| IBIS file stm32u595_599_5a5_5a9_wlcsp150_dsi_smps.ibs
[IBIS ver] 4.2
[File name] stm32u595_599_5a5_5a9_wlcsp150_dsi_smps.ibs
[File Rev] rev2.0
[Date]  11-09-2023
[Source] Data Created at STMicroelectronics
[Notes]  File originated from ELDO simulations.
[Disclaimer]  This information is for modeling purpose only and is
   not guaranteed. The information is subject to change without
   notice.
[Copyright] Copyright 2023 STMicroelectronics Inc.
|   Component stm32u595_599_5a5_5a9_wlcsp150_dsi_smps
[Component] stm32u595_599_5a5_5a9_wlcsp150_dsi_smps
[Manufacturer] STMicroelectronics
[Package]
| variable   typ   min   max
R_pkg  0  NA  NA
L_pkg  0  NA  NA
C_pkg  0  NA  NA
[Pin]   signal_name   model_name
A1  VDDUSB  power
A3  VDD  power
A5  PC12  io8_166m_hslv_ft
A7  VDD  power
A9  PB5  io8_166m_hslv_ft
A11  VDD  power
A13  PC14-OSC32_IN  nc
AA1  VSS  gnd
AA3  PB12  io8_166m_hslv_ft
AA5  PB11  io8_100m_hslv_ft
AA7  PE8  io8_100m_hslv_ft
AA9  PF13  io8_100m_hslv_ft
AA11  PA5  io8_100m_ft
AA13  VSSA_VREFM  nc
AB2  VDD11  nc
AB4  VDDSMPS  nc
AB6  PE13  io8_100m_hslv_ft
AB8  VSS  gnd
AB10  VSS  gnd
AB12  VREFP  nc
AC1  VDD  power
AC3  VSSSMPS  nc
AC5  VLXSMPS  nc
AC7  VDD  power
AC9  VDD  power
AC11  VDD  power
AC13  VDDA  nc
B2  VDD11  nc
B4  PA15  nc
B6  PD4  io8_100m_hslv_ft
B8  PB3  io8_100m_i2c_ft
B10  VDD11  nc
B12  PC15-OSC32_OUT  nc
C1  PA12  io8_100m_ft
C3  VSS  gnd
C5  PD0  io8_100m_hslv_ft
C7  VSS  gnd
C9  PB8  io8_100m_i2c_ft
C11  VSS  gnd
C13  VBAT  power
D2  VSS  gnd
D4  PC10  io8_100m_ft
D6  PD5  io8_100m_hslv_ft
D8  PB6  io8_100m_i2c_ft
D10  PE2  io8_100m_hslv_ft
D12  PE6  io8_100m_hslv_tamp_ft
E1  PA11  io8_100m_ft
E3  PA13  io8_100m_ft
E5  PD1  io8_100m_hslv_ft
E7  PB4  io8_100m_i2c_ft
E9  PE1  io8_100m_hslv_ft
E11  PC13  io8_100m_ft
E13  DSI_D0P  nc
F2  PA9  io8_100m_usb_vbus_ft
F4  PA14  io8_100m_ft
F6  PD6  io8_166m_hslv_ft
F8  PB9  io8_100m_i2c_ft
F10  PE5  io8_100m_hslv_tamp_ft
F12  PF2  io8_100m_hslv_ft
G1  VDDIO2  power
G3  PA10  io8_100m_usb_id
G5  PD2  io8_100m_ft
G7  PB7  io8_spi_hslv_ft
G9  PE3  io8_100m_hslv_tamp_ft
G11  PF0  io8_100m_hslv_ft
G13  DSI_D0N  nc
H2  VSS  gnd
H4  PA8  io8_166m_hslv_ft
H6  PD7  io8_100m_hslv_ft
H8  PE0  io8_100m_hslv_ft
H10  PF1  io8_100m_hslv_ft
H12  VDDDSI  nc
J1  PG7  io8_100m_hslv_ft
J3  PC7  io8_100m_ft
J5  PC11  io8_100m_hslv_ft
J7  PH3-BOOT0  nc
J9  PE4  io8_100m_hslv_tamp_ft
J11  PF6  io8_100m_hslv_ft
J13  DSI_CKP  nc
K2  PG8  io8_100m_i2c_ft
K4  PC8  io8_100m_ft
K6  PD3  io8_166m_hslv_ft
K8  PF10  io8_166m_hslv_ft
K10  PF7  io8_100m_hslv_ft
K12  VSSDSI  nc
L1  PG3  io8_100m_hslv_ft
L3  PG5  io8_100m_hslv_ft
L5  PC9  io8_100m_ft
L7  PC1  io8_spi_hslv_ft
L9  PF9  io8_100m_hslv_ft
L11  PF3  io8_100m_hslv_ft
L13  DSI_CKN  nc
M2  PG4  io8_100m_hslv_ft
M4  PG6  io8_100m_hslv_ft
M6  PB2  io8_100m_hslv_tamp_ft
M8  PA4  io8_100m_hslv_ft
M10  PF8  io8_100m_hslv_ft
M12  VDD11DSI  nc
N1  PG2  io8_100m_hslv_ft
N3  PD13  io8_100m_hslv_ft
N5  PC6  io8_100m_ft
N7  PC5  io8_100m_tamp_ft
N9  PA3  io8_166m_hslv_ft
N11  PF4  io8_spi_ft
N13  DSI_D1P  nc
P2  PD14  io8_100m_hslv_ft
P4  PE14  io8_100m_hslv_ft
P6  PG0  io8_100m_hslv_ft
P8  PA7  io8_100m_hslv_ft
P10  PC0  io8_100m_hslv_ft
P12  VSSDSI  nc
R1  PD15  io8_100m_hslv_ft
R3  PD11  io8_100m_hslv_ft
R5  PE10  io8_166m_hslv_ft
R7  PF11  io8_166m_hslv_ft
R9  PA2  io8_100m_hslv_ft
R11  PF5  io8_spi_ft
R13  DSI_D1N  nc
T2  PD12  io8_100m_hslv_ft
T4  PE15  io8_100m_hslv_ft
T6  PE7  io8_100m_hslv_ft
T8  PC4  io8_100m_hslv_ft
T10  PC3  io8_100m_hslv_ft
T12  VSS  gnd
U1  VDD  power
U3  PD9  io8_100m_hslv_ft
U5  PE11  io8_100m_hslv_ft
U7  PF15  io8_100m_hslv_ft
U9  PA6  io8_100m_hslv_ft
U11  NRST  nc
U13  VDD  power
V2  VSS  gnd
V4  PB14  io8_100m_i2c_ft
V6  PE9  io8_166m_hslv_ft
V8  PF12  io8_100m_hslv_ft
V10  PA1  io8_100m_hslv_tamp_ft
V12  PH1-OSC_OUT   nc
W1  PD10  io8_100m_hslv_ft
W3  PD8  io8_100m_hslv_ft
W5  PB10  io8_spi_hslv_ft
W7  PG1  io8_100m_hslv_ft
W9  PB1  io8_100m_hslv_ft
W11  PA0  io8_100m_hslv_tamp_ft
W13  PH0-OSC_IN  nc
Y2  PB15  nc
Y4  PB13  io8_100m_i2c_ft
Y6  PE12  io8_100m_hslv_ft
Y8  PF14  io8_100m_hslv_ft
Y10  PB0  io8_100m_hslv_ft
Y12  PC2  io8_100m_hslv_ft
[Package Model]   481-wlcsp-150-2rdl-dsi-220915
[Pin Mapping]   pulldown_ref   pullup_ref   | Comment
A1  nc  vddusb
A3  nc  vddiom
A5  gndio  vddiom
A7  nc  vddiom
A9  gndio  vddiom
A11  nc  vddiom
A13  nc  nc
AA1  gndio  nc
AA3  gndio  vddiom
AA5  gndio  vddiom
AA7  gndio  vddiom
AA9  gndio  vddiom
AA11  gndio  vddiom
AA13  nc  nc
AB2  nc  nc
AB4  nc  nc
AB6  gndio  vddiom
AB8  gndio  nc
AB10  gndio  nc
AB12  nc  nc
AC1  nc  vddiom
AC3  nc  nc
AC5  nc  nc
AC7  nc  vddiom
AC9  nc  vddiom
AC11  nc  vddiom
AC13  nc  nc
B2  nc  nc
B4  nc  nc
B6  gndio  vddiom
B8  gndio  vddiom
B10  nc  nc
B12  nc  nc
C1  gndio  vddiom  | Depending on IO usage
| C1  gndio  vddusb  | Depending on IO usage
C3  gndio  nc
C5  gndio  vddiom
C7  gndio  nc
C9  gndio  vddiom
C11  gndio  nc
C13  nc  vsw
D2  gndio  nc
D4  gndio  vddiom
D6  gndio  vddiom
D8  gndio  vddiom
D10  gndio  vddiom
D12  gndio  vddiom
E1  gndio  vddiom  | Depending on IO usage
| E1  gndio  vddusb  | Depending on IO usage
E3  gndio  vddiom  | Depending on IO usage
| E3  gndio  vddusb  | Depending on IO usage
E5  gndio  vddiom
E7  gndio  vddiom
E9  gndio  vddiom
E11  gndio  vddiom  | Depending on IO usage
| E11  gndio  vsw  | Depending on IO usage
E13  nc  nc
F2  gndio  vddiom  | Depending on IO usage
| F2  gndio  vddusb  | Depending on IO usage
F4  gndio  vddiom
F6  gndio  vddiom
F8  gndio  vddiom
F10  gndio  vddiom
F12  gndio  vddiom
G1  nc  vddio2
G3  gndio  vddiom  | Depending on IO usage
| G3  gndio  vddusb  | Depending on IO usage
G5  gndio  vddiom
G7  gndio  vddiom
G9  gndio  vddiom
G11  gndio  vddiom
G13  nc  nc
H2  gndio  nc
H4  gndio  vddiom
H6  gndio  vddiom
H8  gndio  vddiom
H10  gndio  vddiom
H12  nc  nc
J1  gndio  vddiom  | Depending on IO usage
| J1  gndio  vddio2  | Depending on IO usage
J3  gndio  vddiom
J5  gndio  vddiom
J7  nc  nc
J9  gndio  vddiom
J11  gndio  vddiom
J13  nc  nc
K2  gndio  vddiom  | Depending on IO usage
| K2  gndio  vddio2  | Depending on IO usage
K4  gndio  vddiom
K6  gndio  vddiom
K8  gndio  vddiom
K10  gndio  vddiom
K12  nc  nc
L1  gndio  vddiom  | Depending on IO usage
| L1  gndio  vddio2  | Depending on IO usage
L3  gndio  vddiom  | Depending on IO usage
| L3  gndio  vddio2  | Depending on IO usage
L5  gndio  vddiom
L7  gndio  vddiom
L9  gndio  vddiom
L11  gndio  vddiom
L13  nc  nc
M2  gndio  vddiom  | Depending on IO usage
| M2  gndio  vddio2  | Depending on IO usage
M4  gndio  vddiom  | Depending on IO usage
| M4  gndio  vddio2  | Depending on IO usage
M6  gndio  vddiom
M8  gndio  vddiom
M10  gndio  vddiom
M12  nc  nc
N1  gndio  vddiom  | Depending on IO usage
| N1  gndio  vddio2  | Depending on IO usage
N3  gndio  vddiom
N5  gndio  vddiom
N7  gndio  vddiom
N9  gndio  vddiom
N11  gndio  vddiom
N13  nc  nc
P2  gndio  vddiom
P4  gndio  vddiom
P6  gndio  vddiom
P8  gndio  vddiom
P10  gndio  vddiom
P12  nc  nc
R1  gndio  vddiom
R3  gndio  vddiom
R5  gndio  vddiom
R7  gndio  vddiom
R9  gndio  vddiom
R11  gndio  vddiom
R13  nc  nc
T2  gndio  vddiom
T4  gndio  vddiom
T6  gndio  vddiom
T8  gndio  vddiom
T10  gndio  vddiom
T12  gndio  nc
U1  nc  vddiom
U3  gndio  vddiom
U5  gndio  vddiom
U7  gndio  vddiom
U9  gndio  vddiom
U11  nc  nc
U13  nc  vddiom
V2  gndio  nc
V4  gndio  vddiom
V6  gndio  vddiom
V8  gndio  vddiom
V10  gndio  vddiom
V12  nc  nc
W1  gndio  vddiom
W3  gndio  vddiom
W5  gndio  vddiom
W7  gndio  vddiom
W9  gndio  vddiom
W11  gndio  vddiom
W13  nc  nc
Y2  nc  nc
Y4  gndio  vddiom
Y6  gndio  vddiom
Y8  gndio  vddiom
Y10  gndio  vddiom
Y12  gndio  vddiom
[Model Selector] io8_100m_ft
io8_100m_ft_hs_1v2  "IO8_FT 100MHz high speed @ 1.2V"
io8_100m_ft_fs_1v2  "IO8_FT 100MHz fast speed @ 1.2V"
io8_100m_ft_fs_pd_1v2  "IO8_FT 100MHz fast speed @ 1.2V pulldown"
io8_100m_ft_ms_1v2  "IO8_FT 100MHz med speed @ 1.2V"
io8_100m_ft_ms_pd_1v2  "IO8_FT 100MHz med speed @ 1.2V pulldown"
io8_100m_ft_ls_1v2  "IO8_FT 100MHz low speed @ 1.2V"
io8_100m_ft_ls_pd_1v2  "IO8_FT 100MHz low speed @ 1.2V pulldown"
io8_100m_ft_hs_1v8  "IO8_FT 100MHz high speed @ 1.8V"
io8_100m_ft_hs_pd_1v8  "IO8_FT 100MHz high speed @ 1.8V pulldown"
io8_100m_ft_fs_1v8  "IO8_FT 100MHz fast speed @ 1.8V"
io8_100m_ft_fs_pd_1v8  "IO8_FT 100MHz fast speed @ 1.8V pulldown"
io8_100m_ft_ms_1v8  "IO8_FT 100MHz med speed @ 1.8V"
io8_100m_ft_ms_pd_1v8  "IO8_FT 100MHz med speed @ 1.8V pulldown"
io8_100m_ft_ls_1v8  "IO8_FT 100MHz low speed @ 1.8V"
io8_100m_ft_ls_pd_1v8  "IO8_FT 100MHz low speed @ 1.8V pulldown"
io8_100m_ft_hs_3v3  "IO8_FT 100MHz high speed @ 3.3V"
io8_100m_ft_hs_pd_3v3  "IO8_FT 100MHz high speed @ 3.3V pulldown"
io8_100m_ft_fs_3v3  "IO8_FT 100MHz fast speed @ 3.3V"
io8_100m_ft_fs_pd_3v3  "IO8_FT 100MHz fast speed @ 3.3V pulldown"
io8_100m_ft_ms_3v3  "IO8_FT 100MHz med speed @ 3.3V"
io8_100m_ft_ms_pd_3v3  "IO8_FT 100MHz med speed @ 3.3V pulldown"
io8_100m_ft_ls_3v3  "IO8_FT 100MHz low speed @ 3.3V"
io8_100m_ft_ls_pd_3v3  "IO8_FT 100MHz low speed @ 3.3V pulldown"
[Model Selector] io8_100m_hslv_ft
io8_100m_ft_hs_1v2  "IO8_FT 100MHz high speed @ 1.2V"
io8_100m_ft_hs_pu_1v2  "IO8_FT 100MHz high speed @ 1.2V pullup"
io8_100m_ft_hs_pd_1v2  "IO8_FT 100MHz high speed @ 1.2V pulldown"
io8_100m_ft_fs_1v2  "IO8_FT 100MHz fast speed @ 1.2V"
io8_100m_ft_fs_pu_1v2  "IO8_FT 100MHz fast speed @ 1.2V pullup"
io8_100m_ft_fs_pd_1v2  "IO8_FT 100MHz fast speed @ 1.2V pulldown"
io8_100m_ft_ms_1v2  "IO8_FT 100MHz med speed @ 1.2V"
io8_100m_ft_ms_pu_1v2  "IO8_FT 100MHz med speed @ 1.2V pullup"
io8_100m_ft_ms_pd_1v2  "IO8_FT 100MHz med speed @ 1.2V pulldown"
io8_100m_ft_ls_1v2  "IO8_FT 100MHz low speed @ 1.2V"
io8_100m_ft_ls_pu_1v2  "IO8_FT 100MHz low speed @ 1.2V pullup"
io8_100m_ft_ls_pd_1v2  "IO8_FT 100MHz low speed @ 1.2V pulldown"
io8_100m_ft_hs_1v8  "IO8_FT 100MHz high speed @ 1.8V"
io8_100m_ft_hs_pu_1v8  "IO8_FT 100MHz high speed @ 1.8V pullup"
io8_100m_ft_hs_pd_1v8  "IO8_FT 100MHz high speed @ 1.8V pulldown"
io8_100m_ft_fs_1v8  "IO8_FT 100MHz fast speed @ 1.8V"
io8_100m_ft_fs_pu_1v8  "IO8_FT 100MHz fast speed @ 1.8V pullup"
io8_100m_ft_fs_pd_1v8  "IO8_FT 100MHz fast speed @ 1.8V pulldown"
io8_100m_ft_ms_1v8  "IO8_FT 100MHz med speed @ 1.8V"
io8_100m_ft_ms_pu_1v8  "IO8_FT 100MHz med speed @ 1.8V pullup"
io8_100m_ft_ms_pd_1v8  "IO8_FT 100MHz med speed @ 1.8V pulldown"
io8_100m_ft_ls_1v8  "IO8_FT 100MHz low speed @ 1.8V"
io8_100m_ft_ls_pu_1v8  "IO8_FT 100MHz low speed @ 1.8V pullup"
io8_100m_ft_ls_pd_1v8  "IO8_FT 100MHz low speed @ 1.8V pulldown"
io8_100m_ft_hs_3v3  "IO8_FT 100MHz high speed @ 3.3V"
io8_100m_ft_hs_pu_3v3  "IO8_FT 100MHz high speed @ 3.3V pullup"
io8_100m_ft_hs_pd_3v3  "IO8_FT 100MHz high speed @ 3.3V pulldown"
io8_100m_ft_fs_3v3  "IO8_FT 100MHz fast speed @ 3.3V"
io8_100m_ft_fs_pu_3v3  "IO8_FT 100MHz fast speed @ 3.3V pullup"
io8_100m_ft_fs_pd_3v3  "IO8_FT 100MHz fast speed @ 3.3V pulldown"
io8_100m_ft_ms_3v3  "IO8_FT 100MHz med speed @ 3.3V"
io8_100m_ft_ms_pu_3v3  "IO8_FT 100MHz med speed @ 3.3V pullup"
io8_100m_ft_ms_pd_3v3  "IO8_FT 100MHz med speed @ 3.3V pulldown"
io8_100m_ft_ls_3v3  "IO8_FT 100MHz low speed @ 3.3V"
io8_100m_ft_ls_pu_3v3  "IO8_FT 100MHz low speed @ 3.3V pullup"
io8_100m_ft_ls_pd_3v3  "IO8_FT 100MHz low speed @ 3.3V pulldown"
io8_100m_hslv_ft_hs_1v2  "IO8_FT 100MHz HSLV high speed @ 1.2V"
io8_100m_hslv_ft_hs_pu_1v2  "IO8_FT 100MHz HSLV high speed @ 1.2V pullup"
io8_100m_hslv_ft_hs_pd_1v2  "IO8_FT 100MHz HSLV high speed @ 1.2V pulldown"
io8_100m_hslv_ft_fs_1v2  "IO8_FT 100MHz HSLV fast speed @ 1.2V"
io8_100m_hslv_ft_fs_pu_1v2  "IO8_FT 100MHz HSLV fast speed @ 1.2V pullup"
io8_100m_hslv_ft_fs_pd_1v2  "IO8_FT 100MHz HSLV fast speed @ 1.2V pulldown"
io8_100m_hslv_ft_ms_1v2  "IO8_FT 100MHz HSLV med speed @ 1.2V"
io8_100m_hslv_ft_ms_pu_1v2  "IO8_FT 100MHz HSLV med speed @ 1.2V pullup"
io8_100m_hslv_ft_ms_pd_1v2  "IO8_FT 100MHz HSLV med speed @ 1.2V pulldown"
io8_100m_hslv_ft_ls_1v2  "IO8_FT 100MHz HSLV low speed @ 1.2V"
io8_100m_hslv_ft_ls_pu_1v2  "IO8_FT 100MHz HSLV low speed @ 1.2V pullup"
io8_100m_hslv_ft_ls_pd_1v2  "IO8_FT 100MHz HSLV low speed @ 1.2V pulldown"
io8_100m_hslv_ft_hs_1v8  "IO8_FT 100MHz HSLV high speed @ 1.8V"
io8_100m_hslv_ft_hs_pu_1v8  "IO8_FT 100MHz HSLV high speed @ 1.8V pullup"
io8_100m_hslv_ft_hs_pd_1v8  "IO8_FT 100MHz HSLV high speed @ 1.8V pulldown"
io8_100m_hslv_ft_fs_1v8  "IO8_FT 100MHz HSLV fast speed @ 1.8V"
io8_100m_hslv_ft_fs_pu_1v8  "IO8_FT 100MHz HSLV fast speed @ 1.8V pullup"
io8_100m_hslv_ft_fs_pd_1v8  "IO8_FT 100MHz HSLV fast speed @ 1.8V pulldown"
io8_100m_hslv_ft_ms_1v8  "IO8_FT 100MHz HSLV med speed @ 1.8V"
io8_100m_hslv_ft_ms_pu_1v8  "IO8_FT 100MHz HSLV med speed @ 1.8V pullup"
io8_100m_hslv_ft_ms_pd_1v8  "IO8_FT 100MHz HSLV med speed @ 1.8V pulldown"
io8_100m_hslv_ft_ls_1v8  "IO8_FT 100MHz HSLV low speed @ 1.8V"
io8_100m_hslv_ft_ls_pu_1v8  "IO8_FT 100MHz HSLV low speed @ 1.8V pullup"
io8_100m_hslv_ft_ls_pd_1v8  "IO8_FT 100MHz HSLV low speed @ 1.8V pulldown"
io8_100m_hslv_ft_hs_2v5  "IO8_FT 100MHz HSLV high speed @ 2.5V"
io8_100m_hslv_ft_hs_pu_2v5  "IO8_FT 100MHz HSLV high speed @ 2.5V pullup"
io8_100m_hslv_ft_hs_pd_2v5  "IO8_FT 100MHz HSLV high speed @ 2.5V pulldown"
io8_100m_hslv_ft_fs_2v5  "IO8_FT 100MHz HSLV fast speed @ 2.5V"
io8_100m_hslv_ft_fs_pu_2v5  "IO8_FT 100MHz HSLV fast speed @ 2.5V pullup"
io8_100m_hslv_ft_fs_pd_2v5  "IO8_FT 100MHz HSLV fast speed @ 2.5V pulldown"
io8_100m_hslv_ft_ms_2v5  "IO8_FT 100MHz HSLV med speed @ 2.5V"
io8_100m_hslv_ft_ms_pu_2v5  "IO8_FT 100MHz HSLV med speed @ 2.5V pullup"
io8_100m_hslv_ft_ms_pd_2v5  "IO8_FT 100MHz HSLV med speed @ 2.5V pulldown"
io8_100m_hslv_ft_ls_2v5  "IO8_FT 100MHz HSLV low speed @ 2.5V"
io8_100m_hslv_ft_ls_pu_2v5  "IO8_FT 100MHz HSLV low speed @ 2.5V pullup"
io8_100m_hslv_ft_ls_pd_2v5  "IO8_FT 100MHz HSLV low speed @ 2.5V pulldown"
[Model Selector] io8_100m_hslv_tamp_ft
io8_100m_ft_hs_1v2  "IO8_FT 100MHz high speed @ 1.2V"
io8_100m_ft_hs_pu_1v2  "IO8_FT 100MHz high speed @ 1.2V pullup"
io8_100m_ft_hs_pd_1v2  "IO8_FT 100MHz high speed @ 1.2V pulldown"
io8_100m_ft_fs_1v2  "IO8_FT 100MHz fast speed @ 1.2V"
io8_100m_ft_fs_pu_1v2  "IO8_FT 100MHz fast speed @ 1.2V pullup"
io8_100m_ft_fs_pd_1v2  "IO8_FT 100MHz fast speed @ 1.2V pulldown"
io8_100m_ft_ms_1v2  "IO8_FT 100MHz med speed @ 1.2V"
io8_100m_ft_ms_pu_1v2  "IO8_FT 100MHz med speed @ 1.2V pullup"
io8_100m_ft_ms_pd_1v2  "IO8_FT 100MHz med speed @ 1.2V pulldown"
io8_100m_ft_ls_1v2  "IO8_FT 100MHz low speed @ 1.2V"
io8_100m_ft_ls_pu_1v2  "IO8_FT 100MHz low speed @ 1.2V pullup"
io8_100m_ft_ls_pd_1v2  "IO8_FT 100MHz low speed @ 1.2V pulldown"
io8_100m_ft_hs_1v8  "IO8_FT 100MHz high speed @ 1.8V"
io8_100m_ft_hs_pu_1v8  "IO8_FT 100MHz high speed @ 1.8V pullup"
io8_100m_ft_hs_pd_1v8  "IO8_FT 100MHz high speed @ 1.8V pulldown"
io8_100m_ft_fs_1v8  "IO8_FT 100MHz fast speed @ 1.8V"
io8_100m_ft_fs_pu_1v8  "IO8_FT 100MHz fast speed @ 1.8V pullup"
io8_100m_ft_fs_pd_1v8  "IO8_FT 100MHz fast speed @ 1.8V pulldown"
io8_100m_ft_ms_1v8  "IO8_FT 100MHz med speed @ 1.8V"
io8_100m_ft_ms_pu_1v8  "IO8_FT 100MHz med speed @ 1.8V pullup"
io8_100m_ft_ms_pd_1v8  "IO8_FT 100MHz med speed @ 1.8V pulldown"
io8_100m_ft_ls_1v8  "IO8_FT 100MHz low speed @ 1.8V"
io8_100m_ft_ls_pu_1v8  "IO8_FT 100MHz low speed @ 1.8V pullup"
io8_100m_ft_ls_pd_1v8  "IO8_FT 100MHz low speed @ 1.8V pulldown"
io8_100m_ft_hs_3v3  "IO8_FT 100MHz high speed @ 3.3V"
io8_100m_ft_hs_pu_3v3  "IO8_FT 100MHz high speed @ 3.3V pullup"
io8_100m_ft_hs_pd_3v3  "IO8_FT 100MHz high speed @ 3.3V pulldown"
io8_100m_ft_fs_3v3  "IO8_FT 100MHz fast speed @ 3.3V"
io8_100m_ft_fs_pu_3v3  "IO8_FT 100MHz fast speed @ 3.3V pullup"
io8_100m_ft_fs_pd_3v3  "IO8_FT 100MHz fast speed @ 3.3V pulldown"
io8_100m_ft_ms_3v3  "IO8_FT 100MHz med speed @ 3.3V"
io8_100m_ft_ms_pu_3v3  "IO8_FT 100MHz med speed @ 3.3V pullup"
io8_100m_ft_ms_pd_3v3  "IO8_FT 100MHz med speed @ 3.3V pulldown"
io8_100m_ft_ls_3v3  "IO8_FT 100MHz low speed @ 3.3V"
io8_100m_ft_ls_pu_3v3  "IO8_FT 100MHz low speed @ 3.3V pullup"
io8_100m_ft_ls_pd_3v3  "IO8_FT 100MHz low speed @ 3.3V pulldown"
io8_100m_hslv_ft_hs_1v2  "IO8_FT 100MHz HSLV high speed @ 1.2V"
io8_100m_hslv_ft_hs_pu_1v2  "IO8_FT 100MHz HSLV high speed @ 1.2V pullup"
io8_100m_hslv_ft_hs_pd_1v2  "IO8_FT 100MHz HSLV high speed @ 1.2V pulldown"
io8_100m_hslv_ft_fs_1v2  "IO8_FT 100MHz HSLV fast speed @ 1.2V"
io8_100m_hslv_ft_fs_pu_1v2  "IO8_FT 100MHz HSLV fast speed @ 1.2V pullup"
io8_100m_hslv_ft_fs_pd_1v2  "IO8_FT 100MHz HSLV fast speed @ 1.2V pulldown"
io8_100m_hslv_ft_ms_1v2  "IO8_FT 100MHz HSLV med speed @ 1.2V"
io8_100m_hslv_ft_ms_pu_1v2  "IO8_FT 100MHz HSLV med speed @ 1.2V pullup"
io8_100m_hslv_ft_ms_pd_1v2  "IO8_FT 100MHz HSLV med speed @ 1.2V pulldown"
io8_100m_hslv_ft_ls_1v2  "IO8_FT 100MHz HSLV low speed @ 1.2V"
io8_100m_hslv_ft_ls_pu_1v2  "IO8_FT 100MHz HSLV low speed @ 1.2V pullup"
io8_100m_hslv_ft_ls_pd_1v2  "IO8_FT 100MHz HSLV low speed @ 1.2V pulldown"
io8_100m_hslv_ft_hs_1v8  "IO8_FT 100MHz HSLV high speed @ 1.8V"
io8_100m_hslv_ft_hs_pu_1v8  "IO8_FT 100MHz HSLV high speed @ 1.8V pullup"
io8_100m_hslv_ft_hs_pd_1v8  "IO8_FT 100MHz HSLV high speed @ 1.8V pulldown"
io8_100m_hslv_ft_fs_1v8  "IO8_FT 100MHz HSLV fast speed @ 1.8V"
io8_100m_hslv_ft_fs_pu_1v8  "IO8_FT 100MHz HSLV fast speed @ 1.8V pullup"
io8_100m_hslv_ft_fs_pd_1v8  "IO8_FT 100MHz HSLV fast speed @ 1.8V pulldown"
io8_100m_hslv_ft_ms_1v8  "IO8_FT 100MHz HSLV med speed @ 1.8V"
io8_100m_hslv_ft_ms_pu_1v8  "IO8_FT 100MHz HSLV med speed @ 1.8V pullup"
io8_100m_hslv_ft_ms_pd_1v8  "IO8_FT 100MHz HSLV med speed @ 1.8V pulldown"
io8_100m_hslv_ft_ls_1v8  "IO8_FT 100MHz HSLV low speed @ 1.8V"
io8_100m_hslv_ft_ls_pu_1v8  "IO8_FT 100MHz HSLV low speed @ 1.8V pullup"
io8_100m_hslv_ft_ls_pd_1v8  "IO8_FT 100MHz HSLV low speed @ 1.8V pulldown"
io8_100m_hslv_ft_hs_2v5  "IO8_FT 100MHz HSLV high speed @ 2.5V"
io8_100m_hslv_ft_hs_pu_2v5  "IO8_FT 100MHz HSLV high speed @ 2.5V pullup"
io8_100m_hslv_ft_hs_pd_2v5  "IO8_FT 100MHz HSLV high speed @ 2.5V pulldown"
io8_100m_hslv_ft_fs_2v5  "IO8_FT 100MHz HSLV fast speed @ 2.5V"
io8_100m_hslv_ft_fs_pu_2v5  "IO8_FT 100MHz HSLV fast speed @ 2.5V pullup"
io8_100m_hslv_ft_fs_pd_2v5  "IO8_FT 100MHz HSLV fast speed @ 2.5V pulldown"
io8_100m_hslv_ft_ms_2v5  "IO8_FT 100MHz HSLV med speed @ 2.5V"
io8_100m_hslv_ft_ms_pu_2v5  "IO8_FT 100MHz HSLV med speed @ 2.5V pullup"
io8_100m_hslv_ft_ms_pd_2v5  "IO8_FT 100MHz HSLV med speed @ 2.5V pulldown"
io8_100m_hslv_ft_ls_2v5  "IO8_FT 100MHz HSLV low speed @ 2.5V"
io8_100m_hslv_ft_ls_pu_2v5  "IO8_FT 100MHz HSLV low speed @ 2.5V pullup"
io8_100m_hslv_ft_ls_pd_2v5  "IO8_FT 100MHz HSLV low speed @ 2.5V pulldown"
io8_ft_v33_hs_1v2  "IO8_FT_V33 high speed @ 1.2V"
io8_ft_v33_hs_pu_1v2  "IO8_FT_V33 high speed @ 1.2V pullup"
io8_ft_v33_hs_pd_1v2  "IO8_FT_V33 high speed @ 1.2V pulldown"
io8_ft_v33_fs_1v2  "IO8_FT_V33 fast speed @ 1.2V"
io8_ft_v33_fs_pu_1v2  "IO8_FT_V33 fast speed @ 1.2V pullup"
io8_ft_v33_fs_pd_1v2  "IO8_FT_V33 fast speed @ 1.2V pulldown"
io8_ft_v33_ms_1v2  "IO8_FT_V33 med speed @ 1.2V"
io8_ft_v33_ms_pu_1v2  "IO8_FT_V33 med speed @ 1.2V pullup"
io8_ft_v33_ms_pd_1v2  "IO8_FT_V33 med speed @ 1.2V pulldown"
io8_ft_v33_ls_1v2  "IO8_FT_V33 low speed @ 1.2V"
io8_ft_v33_ls_pu_1v2  "IO8_FT_V33 low speed @ 1.2V pullup"
io8_ft_v33_ls_pd_1v2  "IO8_FT_V33 low speed @ 1.2V pulldown"
io8_ft_v33_hs_1v8  "IO8_FT_V33 high speed @ 1.8V"
io8_ft_v33_hs_pu_1v8  "IO8_FT_V33 high speed @ 1.8V pullup"
io8_ft_v33_hs_pd_1v8  "IO8_FT_V33 high speed @ 1.8V pulldown"
io8_ft_v33_fs_1v8  "IO8_FT_V33 fast speed @ 1.8V"
io8_ft_v33_fs_pu_1v8  "IO8_FT_V33 fast speed @ 1.8V pullup"
io8_ft_v33_fs_pd_1v8  "IO8_FT_V33 fast speed @ 1.8V pulldown"
io8_ft_v33_ms_1v8  "IO8_FT_V33 med speed @ 1.8V"
io8_ft_v33_ms_pu_1v8  "IO8_FT_V33 med speed @ 1.8V pullup"
io8_ft_v33_ms_pd_1v8  "IO8_FT_V33 med speed @ 1.8V pulldown"
io8_ft_v33_ls_1v8  "IO8_FT_V33 low speed @ 1.8V"
io8_ft_v33_ls_pu_1v8  "IO8_FT_V33 low speed @ 1.8V pullup"
io8_ft_v33_ls_pd_1v8  "IO8_FT_V33 low speed @ 1.8V pulldown"
io8_ft_v33_hs_3v3  "IO8_FT_V33 high speed @ 3.3V"
io8_ft_v33_hs_pu_3v3  "IO8_FT_V33 high speed @ 3.3V pullup"
io8_ft_v33_hs_pd_3v3  "IO8_FT_V33 high speed @ 3.3V pulldown"
io8_ft_v33_fs_3v3  "IO8_FT_V33 fast speed @ 3.3V"
io8_ft_v33_fs_pu_3v3  "IO8_FT_V33 fast speed @ 3.3V pullup"
io8_ft_v33_fs_pd_3v3  "IO8_FT_V33 fast speed @ 3.3V pulldown"
io8_ft_v33_ms_3v3  "IO8_FT_V33 med speed @ 3.3V"
io8_ft_v33_ms_pu_3v3  "IO8_FT_V33 med speed @ 3.3V pullup"
io8_ft_v33_ms_pd_3v3  "IO8_FT_V33 med speed @ 3.3V pulldown"
io8_ft_v33_ls_3v3  "IO8_FT_V33 low speed @ 3.3V"
io8_ft_v33_ls_pu_3v3  "IO8_FT_V33 low speed @ 3.3V pullup"
io8_ft_v33_ls_pd_3v3  "IO8_FT_V33 low speed @ 3.3V pulldown"
[Model Selector] io8_100m_i2c_ft
io8_100m_ft_hs_1v2  "IO8_FT 100MHz high speed @ 1.2V"
io8_100m_ft_hs_pu_1v2  "IO8_FT 100MHz high speed @ 1.2V pullup"
io8_100m_ft_hs_pd_1v2  "IO8_FT 100MHz high speed @ 1.2V pulldown"
io8_100m_ft_fs_1v2  "IO8_FT 100MHz fast speed @ 1.2V"
io8_100m_ft_fs_pu_1v2  "IO8_FT 100MHz fast speed @ 1.2V pullup"
io8_100m_ft_fs_pd_1v2  "IO8_FT 100MHz fast speed @ 1.2V pulldown"
io8_100m_ft_ms_1v2  "IO8_FT 100MHz med speed @ 1.2V"
io8_100m_ft_ms_pu_1v2  "IO8_FT 100MHz med speed @ 1.2V pullup"
io8_100m_ft_ms_pd_1v2  "IO8_FT 100MHz med speed @ 1.2V pulldown"
io8_100m_ft_ls_1v2  "IO8_FT 100MHz low speed @ 1.2V"
io8_100m_ft_ls_pu_1v2  "IO8_FT 100MHz low speed @ 1.2V pullup"
io8_100m_ft_ls_pd_1v2  "IO8_FT 100MHz low speed @ 1.2V pulldown"
io8_100m_ft_hs_1v8  "IO8_FT 100MHz high speed @ 1.8V"
io8_100m_ft_hs_pu_1v8  "IO8_FT 100MHz high speed @ 1.8V pullup"
io8_100m_ft_hs_pd_1v8  "IO8_FT 100MHz high speed @ 1.8V pulldown"
io8_100m_ft_fs_1v8  "IO8_FT 100MHz fast speed @ 1.8V"
io8_100m_ft_fs_pu_1v8  "IO8_FT 100MHz fast speed @ 1.8V pullup"
io8_100m_ft_fs_pd_1v8  "IO8_FT 100MHz fast speed @ 1.8V pulldown"
io8_100m_ft_ms_1v8  "IO8_FT 100MHz med speed @ 1.8V"
io8_100m_ft_ms_pu_1v8  "IO8_FT 100MHz med speed @ 1.8V pullup"
io8_100m_ft_ms_pd_1v8  "IO8_FT 100MHz med speed @ 1.8V pulldown"
io8_100m_ft_ls_1v8  "IO8_FT 100MHz low speed @ 1.8V"
io8_100m_ft_ls_pu_1v8  "IO8_FT 100MHz low speed @ 1.8V pullup"
io8_100m_ft_ls_pd_1v8  "IO8_FT 100MHz low speed @ 1.8V pulldown"
io8_100m_ft_hs_3v3  "IO8_FT 100MHz high speed @ 3.3V"
io8_100m_ft_hs_pu_3v3  "IO8_FT 100MHz high speed @ 3.3V pullup"
io8_100m_ft_hs_pd_3v3  "IO8_FT 100MHz high speed @ 3.3V pulldown"
io8_100m_ft_fs_3v3  "IO8_FT 100MHz fast speed @ 3.3V"
io8_100m_ft_fs_pu_3v3  "IO8_FT 100MHz fast speed @ 3.3V pullup"
io8_100m_ft_fs_pd_3v3  "IO8_FT 100MHz fast speed @ 3.3V pulldown"
io8_100m_ft_ms_3v3  "IO8_FT 100MHz med speed @ 3.3V"
io8_100m_ft_ms_pu_3v3  "IO8_FT 100MHz med speed @ 3.3V pullup"
io8_100m_ft_ms_pd_3v3  "IO8_FT 100MHz med speed @ 3.3V pulldown"
io8_100m_ft_ls_3v3  "IO8_FT 100MHz low speed @ 3.3V"
io8_100m_ft_ls_pu_3v3  "IO8_FT 100MHz low speed @ 3.3V pullup"
io8_100m_ft_ls_pd_3v3  "IO8_FT 100MHz low speed @ 3.3V pulldown"
io8_100m_i2c_ft_1v2  "IO8_FT 100MHz I2C @ 1.2V"
io8_100m_i2c_ft_pu_1v2  "IO8_FT 100MHz I2C @ 1.2V pullup"
io8_100m_i2c_ft_pd_1v2  "IO8_FT 100MHz I2C @ 1.2V pulldown"
io8_100m_i2c_ft_1v8  "IO8_FT 100MHz I2C @ 1.8V"
io8_100m_i2c_ft_pu_1v8  "IO8_FT 100MHz I2C @ 1.8V pullup"
io8_100m_i2c_ft_pd_1v8  "IO8_FT 100MHz I2C @ 1,8V pulldown"
io8_100m_i2c_ft_3v3  "IO8_FT 100MHz I2C @ 3.3V"
io8_100m_i2c_ft_pu_3v3  "IO8_FT 100MHz I2C HSLV @ 3.3V pullup"
io8_100m_i2c_ft_pd_3v3  "IO8_FT 100MHz I2C @ 3.3V pulldown"
[Model Selector] io8_100m_tamp_ft
io8_100m_ft_hs_1v2  "IO8_FT 100MHz high speed @ 1.2V"
io8_100m_ft_hs_pu_1v2  "IO8_FT 100MHz high speed @ 1.2V pullup"
io8_100m_ft_hs_pd_1v2  "IO8_FT 100MHz high speed @ 1.2V pulldown"
io8_100m_ft_fs_1v2  "IO8_FT 100MHz fast speed @ 1.2V"
io8_100m_ft_fs_pu_1v2  "IO8_FT 100MHz fast speed @ 1.2V pullup"
io8_100m_ft_fs_pd_1v2  "IO8_FT 100MHz fast speed @ 1.2V pulldown"
io8_100m_ft_ms_1v2  "IO8_FT 100MHz med speed @ 1.2V"
io8_100m_ft_ms_pu_1v2  "IO8_FT 100MHz med speed @ 1.2V pullup"
io8_100m_ft_ms_pd_1v2  "IO8_FT 100MHz med speed @ 1.2V pulldown"
io8_100m_ft_ls_1v2  "IO8_FT 100MHz low speed @ 1.2V"
io8_100m_ft_ls_pu_1v2  "IO8_FT 100MHz low speed @ 1.2V pullup"
io8_100m_ft_ls_pd_1v2  "IO8_FT 100MHz low speed @ 1.2V pulldown"
io8_100m_ft_hs_1v8  "IO8_FT 100MHz high speed @ 1.8V"
io8_100m_ft_hs_pu_1v8  "IO8_FT 100MHz high speed @ 1.8V pullup"
io8_100m_ft_hs_pd_1v8  "IO8_FT 100MHz high speed @ 1.8V pulldown"
io8_100m_ft_fs_1v8  "IO8_FT 100MHz fast speed @ 1.8V"
io8_100m_ft_fs_pu_1v8  "IO8_FT 100MHz fast speed @ 1.8V pullup"
io8_100m_ft_fs_pd_1v8  "IO8_FT 100MHz fast speed @ 1.8V pulldown"
io8_100m_ft_ms_1v8  "IO8_FT 100MHz med speed @ 1.8V"
io8_100m_ft_ms_pu_1v8  "IO8_FT 100MHz med speed @ 1.8V pullup"
io8_100m_ft_ms_pd_1v8  "IO8_FT 100MHz med speed @ 1.8V pulldown"
io8_100m_ft_ls_1v8  "IO8_FT 100MHz low speed @ 1.8V"
io8_100m_ft_ls_pu_1v8  "IO8_FT 100MHz low speed @ 1.8V pullup"
io8_100m_ft_ls_pd_1v8  "IO8_FT 100MHz low speed @ 1.8V pulldown"
io8_100m_ft_hs_3v3  "IO8_FT 100MHz high speed @ 3.3V"
io8_100m_ft_hs_pu_3v3  "IO8_FT 100MHz high speed @ 3.3V pullup"
io8_100m_ft_hs_pd_3v3  "IO8_FT 100MHz high speed @ 3.3V pulldown"
io8_100m_ft_fs_3v3  "IO8_FT 100MHz fast speed @ 3.3V"
io8_100m_ft_fs_pu_3v3  "IO8_FT 100MHz fast speed @ 3.3V pullup"
io8_100m_ft_fs_pd_3v3  "IO8_FT 100MHz fast speed @ 3.3V pulldown"
io8_100m_ft_ms_3v3  "IO8_FT 100MHz med speed @ 3.3V"
io8_100m_ft_ms_pu_3v3  "IO8_FT 100MHz med speed @ 3.3V pullup"
io8_100m_ft_ms_pd_3v3  "IO8_FT 100MHz med speed @ 3.3V pulldown"
io8_100m_ft_ls_3v3  "IO8_FT 100MHz low speed @ 3.3V"
io8_100m_ft_ls_pu_3v3  "IO8_FT 100MHz low speed @ 3.3V pullup"
io8_100m_ft_ls_pd_3v3  "IO8_FT 100MHz low speed @ 3.3V pulldown"
io8_ft_v33_hs_1v2  "IO8_FT_V33 high speed @ 1.2V"
io8_ft_v33_hs_pu_1v2  "IO8_FT_V33 high speed @ 1.2V pullup"
io8_ft_v33_hs_pd_1v2  "IO8_FT_V33 high speed @ 1.2V pulldown"
io8_ft_v33_fs_1v2  "IO8_FT_V33 fast speed @ 1.2V"
io8_ft_v33_fs_pu_1v2  "IO8_FT_V33 fast speed @ 1.2V pullup"
io8_ft_v33_fs_pd_1v2  "IO8_FT_V33 fast speed @ 1.2V pulldown"
io8_ft_v33_ms_1v2  "IO8_FT_V33 med speed @ 1.2V"
io8_ft_v33_ms_pu_1v2  "IO8_FT_V33 med speed @ 1.2V pullup"
io8_ft_v33_ms_pd_1v2  "IO8_FT_V33 med speed @ 1.2V pulldown"
io8_ft_v33_ls_1v2  "IO8_FT_V33 low speed @ 1.2V"
io8_ft_v33_ls_pu_1v2  "IO8_FT_V33 low speed @ 1.2V pullup"
io8_ft_v33_ls_pd_1v2  "IO8_FT_V33 low speed @ 1.2V pulldown"
io8_ft_v33_hs_1v8  "IO8_FT_V33 high speed @ 1.8V"
io8_ft_v33_hs_pu_1v8  "IO8_FT_V33 high speed @ 1.8V pullup"
io8_ft_v33_hs_pd_1v8  "IO8_FT_V33 high speed @ 1.8V pulldown"
io8_ft_v33_fs_1v8  "IO8_FT_V33 fast speed @ 1.8V"
io8_ft_v33_fs_pu_1v8  "IO8_FT_V33 fast speed @ 1.8V pullup"
io8_ft_v33_fs_pd_1v8  "IO8_FT_V33 fast speed @ 1.8V pulldown"
io8_ft_v33_ms_1v8  "IO8_FT_V33 med speed @ 1.8V"
io8_ft_v33_ms_pu_1v8  "IO8_FT_V33 med speed @ 1.8V pullup"
io8_ft_v33_ms_pd_1v8  "IO8_FT_V33 med speed @ 1.8V pulldown"
io8_ft_v33_ls_1v8  "IO8_FT_V33 low speed @ 1.8V"
io8_ft_v33_ls_pu_1v8  "IO8_FT_V33 low speed @ 1.8V pullup"
io8_ft_v33_ls_pd_1v8  "IO8_FT_V33 low speed @ 1.8V pulldown"
io8_ft_v33_hs_3v3  "IO8_FT_V33 high speed @ 3.3V"
io8_ft_v33_hs_pu_3v3  "IO8_FT_V33 high speed @ 3.3V pullup"
io8_ft_v33_hs_pd_3v3  "IO8_FT_V33 high speed @ 3.3V pulldown"
io8_ft_v33_fs_3v3  "IO8_FT_V33 fast speed @ 3.3V"
io8_ft_v33_fs_pu_3v3  "IO8_FT_V33 fast speed @ 3.3V pullup"
io8_ft_v33_fs_pd_3v3  "IO8_FT_V33 fast speed @ 3.3V pulldown"
io8_ft_v33_ms_3v3  "IO8_FT_V33 med speed @ 3.3V"
io8_ft_v33_ms_pu_3v3  "IO8_FT_V33 med speed @ 3.3V pullup"
io8_ft_v33_ms_pd_3v3  "IO8_FT_V33 med speed @ 3.3V pulldown"
io8_ft_v33_ls_3v3  "IO8_FT_V33 low speed @ 3.3V"
io8_ft_v33_ls_pu_3v3  "IO8_FT_V33 low speed @ 3.3V pullup"
io8_ft_v33_ls_pd_3v3  "IO8_FT_V33 low speed @ 3.3V pulldown"
[Model Selector] io8_100m_usb_id
io8_100m_ft_hs_1v2  "IO8_FT 100MHz high speed @ 1.2V"
io8_100m_ft_hs_pu_1v2  "IO8_FT 100MHz high speed @ 1.2V pullup"
io8_100m_ft_hs_pd_1v2  "IO8_FT 100MHz high speed @ 1.2V pulldown"
io8_100m_ft_fs_1v2  "IO8_FT 100MHz fast speed @ 1.2V"
io8_100m_ft_fs_pu_1v2  "IO8_FT 100MHz fast speed @ 1.2V pullup"
io8_100m_ft_fs_pd_1v2  "IO8_FT 100MHz fast speed @ 1.2V pulldown"
io8_100m_ft_ms_1v2  "IO8_FT 100MHz med speed @ 1.2V"
io8_100m_ft_ms_pu_1v2  "IO8_FT 100MHz med speed @ 1.2V pullup"
io8_100m_ft_ms_pd_1v2  "IO8_FT 100MHz med speed @ 1.2V pulldown"
io8_100m_ft_ls_1v2  "IO8_FT 100MHz low speed @ 1.2V"
io8_100m_ft_ls_pu_1v2  "IO8_FT 100MHz low speed @ 1.2V pullup"
io8_100m_ft_ls_pd_1v2  "IO8_FT 100MHz low speed @ 1.2V pulldown"
io8_100m_ft_hs_1v8  "IO8_FT 100MHz high speed @ 1.8V"
io8_100m_ft_hs_pu_1v8  "IO8_FT 100MHz high speed @ 1.8V pullup"
io8_100m_ft_hs_pd_1v8  "IO8_FT 100MHz high speed @ 1.8V pulldown"
io8_100m_ft_fs_1v8  "IO8_FT 100MHz fast speed @ 1.8V"
io8_100m_ft_fs_pu_1v8  "IO8_FT 100MHz fast speed @ 1.8V pullup"
io8_100m_ft_fs_pd_1v8  "IO8_FT 100MHz fast speed @ 1.8V pulldown"
io8_100m_ft_ms_1v8  "IO8_FT 100MHz med speed @ 1.8V"
io8_100m_ft_ms_pu_1v8  "IO8_FT 100MHz med speed @ 1.8V pullup"
io8_100m_ft_ms_pd_1v8  "IO8_FT 100MHz med speed @ 1.8V pulldown"
io8_100m_ft_ls_1v8  "IO8_FT 100MHz low speed @ 1.8V"
io8_100m_ft_ls_pu_1v8  "IO8_FT 100MHz low speed @ 1.8V pullup"
io8_100m_ft_ls_pd_1v8  "IO8_FT 100MHz low speed @ 1.8V pulldown"
io8_100m_ft_hs_3v3  "IO8_FT 100MHz high speed @ 3.3V"
io8_100m_ft_hs_pu_3v3  "IO8_FT 100MHz high speed @ 3.3V pullup"
io8_100m_ft_hs_pd_3v3  "IO8_FT 100MHz high speed @ 3.3V pulldown"
io8_100m_ft_fs_3v3  "IO8_FT 100MHz fast speed @ 3.3V"
io8_100m_ft_fs_pu_3v3  "IO8_FT 100MHz fast speed @ 3.3V pullup"
io8_100m_ft_fs_pd_3v3  "IO8_FT 100MHz fast speed @ 3.3V pulldown"
io8_100m_ft_ms_3v3  "IO8_FT 100MHz med speed @ 3.3V"
io8_100m_ft_ms_pu_3v3  "IO8_FT 100MHz med speed @ 3.3V pullup"
io8_100m_ft_ms_pd_3v3  "IO8_FT 100MHz med speed @ 3.3V pulldown"
io8_100m_ft_ls_3v3  "IO8_FT 100MHz low speed @ 3.3V"
io8_100m_ft_ls_pu_3v3  "IO8_FT 100MHz low speed @ 3.3V pullup"
io8_100m_ft_ls_pd_3v3  "IO8_FT 100MHz low speed @ 3.3V pulldown"
io8usb_id_nopu  "IOUSB ID @ 3.3V"
io8usb_id_pu  "IOUSB ID @ 3.3V pullup"
[Model Selector] io8_100m_usb_vbus_ft
io8_100m_ft_hs_1v2  "IO8_FT 100MHz high speed @ 1.2V"
io8_100m_ft_hs_pu_1v2  "IO8_FT 100MHz high speed @ 1.2V pullup"
io8_100m_ft_hs_pd_1v2  "IO8_FT 100MHz high speed @ 1.2V pulldown"
io8_100m_ft_fs_1v2  "IO8_FT 100MHz fast speed @ 1.2V"
io8_100m_ft_fs_pu_1v2  "IO8_FT 100MHz fast speed @ 1.2V pullup"
io8_100m_ft_fs_pd_1v2  "IO8_FT 100MHz fast speed @ 1.2V pulldown"
io8_100m_ft_ms_1v2  "IO8_FT 100MHz med speed @ 1.2V"
io8_100m_ft_ms_pu_1v2  "IO8_FT 100MHz med speed @ 1.2V pullup"
io8_100m_ft_ms_pd_1v2  "IO8_FT 100MHz med speed @ 1.2V pulldown"
io8_100m_ft_ls_1v2  "IO8_FT 100MHz low speed @ 1.2V"
io8_100m_ft_ls_pu_1v2  "IO8_FT 100MHz low speed @ 1.2V pullup"
io8_100m_ft_ls_pd_1v2  "IO8_FT 100MHz low speed @ 1.2V pulldown"
io8_100m_ft_hs_1v8  "IO8_FT 100MHz high speed @ 1.8V"
io8_100m_ft_hs_pu_1v8  "IO8_FT 100MHz high speed @ 1.8V pullup"
io8_100m_ft_hs_pd_1v8  "IO8_FT 100MHz high speed @ 1.8V pulldown"
io8_100m_ft_fs_1v8  "IO8_FT 100MHz fast speed @ 1.8V"
io8_100m_ft_fs_pu_1v8  "IO8_FT 100MHz fast speed @ 1.8V pullup"
io8_100m_ft_fs_pd_1v8  "IO8_FT 100MHz fast speed @ 1.8V pulldown"
io8_100m_ft_ms_1v8  "IO8_FT 100MHz med speed @ 1.8V"
io8_100m_ft_ms_pu_1v8  "IO8_FT 100MHz med speed @ 1.8V pullup"
io8_100m_ft_ms_pd_1v8  "IO8_FT 100MHz med speed @ 1.8V pulldown"
io8_100m_ft_ls_1v8  "IO8_FT 100MHz low speed @ 1.8V"
io8_100m_ft_ls_pu_1v8  "IO8_FT 100MHz low speed @ 1.8V pullup"
io8_100m_ft_ls_pd_1v8  "IO8_FT 100MHz low speed @ 1.8V pulldown"
io8_100m_ft_hs_3v3  "IO8_FT 100MHz high speed @ 3.3V"
io8_100m_ft_hs_pu_3v3  "IO8_FT 100MHz high speed @ 3.3V pullup"
io8_100m_ft_hs_pd_3v3  "IO8_FT 100MHz high speed @ 3.3V pulldown"
io8_100m_ft_fs_3v3  "IO8_FT 100MHz fast speed @ 3.3V"
io8_100m_ft_fs_pu_3v3  "IO8_FT 100MHz fast speed @ 3.3V pullup"
io8_100m_ft_fs_pd_3v3  "IO8_FT 100MHz fast speed @ 3.3V pulldown"
io8_100m_ft_ms_3v3  "IO8_FT 100MHz med speed @ 3.3V"
io8_100m_ft_ms_pu_3v3  "IO8_FT 100MHz med speed @ 3.3V pullup"
io8_100m_ft_ms_pd_3v3  "IO8_FT 100MHz med speed @ 3.3V pulldown"
io8_100m_ft_ls_3v3  "IO8_FT 100MHz low speed @ 3.3V"
io8_100m_ft_ls_pu_3v3  "IO8_FT 100MHz low speed @ 3.3V pullup"
io8_100m_ft_ls_pd_3v3  "IO8_FT 100MHz low speed @ 3.3V pulldown"
io8usb_adp "IOUSB ADP @ 3.3V"
io8usb_vbus "IOUSB VBUS @ 3.3V"
[Model Selector] io8_166m_hslv_ft
io8_166m_ft_hs_1v2  "IO8_FT 166MHz high speed @ 1.2V"
io8_166m_ft_hs_pu_1v2  "IO8_FT 166MHz high speed @ 1.2V pullup"
io8_166m_ft_hs_pd_1v2  "IO8_FT 166MHz high speed @ 1.2V pulldown"
io8_166m_ft_fs_1v2  "IO8_FT 166MHz fast speed @ 1.2V"
io8_166m_ft_fs_pu_1v2  "IO8_FT 166MHz fast speed @ 1.2V pullup"
io8_166m_ft_fs_pd_1v2  "IO8_FT 166MHz fast speed @ 1.2V pulldown"
io8_166m_ft_ms_1v2  "IO8_FT 166MHz med speed @ 1.2V"
io8_166m_ft_ms_pu_1v2  "IO8_FT 166MHz med speed @ 1.2V pullup"
io8_166m_ft_ms_pd_1v2  "IO8_FT 166MHz med speed @ 1.2V pulldown"
io8_166m_ft_ls_1v2  "IO8_FT 166MHz low speed @ 1.2V"
io8_166m_ft_ls_pu_1v2  "IO8_FT 166MHz low speed @ 1.2V pullup"
io8_166m_ft_ls_pd_1v2  "IO8_FT 166MHz low speed @ 1.2V pulldown"
io8_166m_ft_hs_1v8  "IO8_FT 166MHz high speed @ 1.8V"
io8_166m_ft_hs_pu_1v8  "IO8_FT 166MHz high speed @ 1.8V pullup"
io8_166m_ft_hs_pd_1v8  "IO8_FT 166MHz high speed @ 1.8V pulldown"
io8_166m_ft_fs_1v8  "IO8_FT 166MHz fast speed @ 1.8V"
io8_166m_ft_fs_pu_1v8  "IO8_FT 166MHz fast speed @ 1.8V pullup"
io8_166m_ft_fs_pd_1v8  "IO8_FT 166MHz fast speed @ 1.8V pulldown"
io8_166m_ft_ms_1v8  "IO8_FT 166MHz med speed @ 1.8V"
io8_166m_ft_ms_pu_1v8  "IO8_FT 166MHz med speed @ 1.8V pullup"
io8_166m_ft_ms_pd_1v8  "IO8_FT 166MHz med speed @ 1.8V pulldown"
io8_166m_ft_ls_1v8  "IO8_FT 166MHz low speed @ 1.8V"
io8_166m_ft_ls_pu_1v8  "IO8_FT 166MHz low speed @ 1.8V pullup"
io8_166m_ft_ls_pd_1v8  "IO8_FT 166MHz low speed @ 1.8V pulldown"
io8_166m_ft_hs_3v3  "IO8_FT 166MHz high speed @ 3.3V"
io8_166m_ft_hs_pu_3v3  "IO8_FT 166MHz high speed @ 3.3V pullup"
io8_166m_ft_hs_pd_3v3  "IO8_FT 166MHz high speed @ 3.3V pulldown"
io8_166m_ft_fs_3v3  "IO8_FT 166MHz fast speed @ 3.3V"
io8_166m_ft_fs_pu_3v3  "IO8_FT 166MHz fast speed @ 3.3V pullup"
io8_166m_ft_fs_pd_3v3  "IO8_FT 166MHz fast speed @ 3.3V pulldown"
io8_166m_ft_ms_3v3  "IO8_FT 166MHz med speed @ 3.3V"
io8_166m_ft_ms_pu_3v3  "IO8_FT 166MHz med speed @ 3.3V pullup"
io8_166m_ft_ms_pd_3v3  "IO8_FT 166MHz med speed @ 3.3V pulldown"
io8_166m_ft_ls_3v3  "IO8_FT 166MHz low speed @ 3.3V"
io8_166m_ft_ls_pu_3v3  "IO8_FT 166MHz low speed @ 3.3V pullup"
io8_166m_ft_ls_pd_3v3  "IO8_FT 166MHz low speed @ 3.3V pulldown"
io8_166m_hslv_ft_hs_1v2  "IO8_FT 166MHz HSLV high speed @ 1.2V"
io8_166m_hslv_ft_hs_pu_1v2  "IO8_FT 166MHz HSLV high speed @ 1.2V pullup"
io8_166m_hslv_ft_hs_pd_1v2  "IO8_FT 166MHz HSLV high speed @ 1.2V pulldown"
io8_166m_hslv_ft_fs_1v2  "IO8_FT 166MHz HSLV fast speed @ 1.2V"
io8_166m_hslv_ft_fs_pu_1v2  "IO8_FT 166MHz HSLV fast speed @ 1.2V pullup"
io8_166m_hslv_ft_fs_pd_1v2  "IO8_FT 166MHz HSLV fast speed @ 1.2V pulldown"
io8_166m_hslv_ft_ms_1v2  "IO8_FT 166MHz HSLV med speed @ 1.2V"
io8_166m_hslv_ft_ms_pu_1v2  "IO8_FT 166MHz HSLV med speed @ 1.2V pullup"
io8_166m_hslv_ft_ms_pd_1v2  "IO8_FT 166MHz HSLV med speed @ 1.2V pulldown"
io8_166m_hslv_ft_ls_1v2  "IO8_FT 166MHz HSLV low speed @ 1.2V"
io8_166m_hslv_ft_ls_pu_1v2  "IO8_FT 166MHz HSLV low speed @ 1.2V pullup"
io8_166m_hslv_ft_ls_pd_1v2  "IO8_FT 166MHz HSLV low speed @ 1.2V pulldown"
io8_166m_hslv_ft_hs_1v8  "IO8_FT 166MHz HSLV high speed @ 1.8V"
io8_166m_hslv_ft_hs_pu_1v8  "IO8_FT 166MHz HSLV high speed @ 1.8V pullup"
io8_166m_hslv_ft_hs_pd_1v8  "IO8_FT 166MHz HSLV high speed @ 1.8V pulldown"
io8_166m_hslv_ft_fs_1v8  "IO8_FT 166MHz HSLV fast speed @ 1.8V"
io8_166m_hslv_ft_fs_pu_1v8  "IO8_FT 166MHz HSLV fast speed @ 1.8V pullup"
io8_166m_hslv_ft_fs_pd_1v8  "IO8_FT 166MHz HSLV fast speed @ 1.8V pulldown"
io8_166m_hslv_ft_ms_1v8  "IO8_FT 166MHz HSLV med speed @ 1.8V"
io8_166m_hslv_ft_ms_pu_1v8  "IO8_FT 166MHz HSLV med speed @ 1.8V pullup"
io8_166m_hslv_ft_ms_pd_1v8  "IO8_FT 166MHz HSLV med speed @ 1.8V pulldown"
io8_166m_hslv_ft_ls_1v8  "IO8_FT 166MHz HSLV low speed @ 1.8V"
io8_166m_hslv_ft_ls_pu_1v8  "IO8_FT 166MHz HSLV low speed @ 1.8V pullup"
io8_166m_hslv_ft_ls_pd_1v8  "IO8_FT 166MHz HSLV low speed @ 1.8V pulldown"
io8_166m_hslv_ft_hs_2v5  "IO8_FT 166MHz HSLV high speed @ 2.5V"
io8_166m_hslv_ft_hs_pu_2v5  "IO8_FT 166MHz HSLV high speed @ 2.5V pullup"
io8_166m_hslv_ft_hs_pd_2v5  "IO8_FT 166MHz HSLV high speed @ 2.5V pulldown"
io8_166m_hslv_ft_fs_2v5  "IO8_FT 166MHz HSLV fast speed @ 2.5V"
io8_166m_hslv_ft_fs_pu_2v5  "IO8_FT 166MHz HSLV fast speed @ 2.5V pullup"
io8_166m_hslv_ft_fs_pd_2v5  "IO8_FT 166MHz HSLV fast speed @ 2.5V pulldown"
io8_166m_hslv_ft_ms_2v5  "IO8_FT 166MHz HSLV med speed @ 2.5V"
io8_166m_hslv_ft_ms_pu_2v5  "IO8_FT 166MHz HSLV med speed @ 2.5V pullup"
io8_166m_hslv_ft_ms_pd_2v5  "IO8_FT 166MHz HSLV med speed @ 2.5V pulldown"
io8_166m_hslv_ft_ls_2v5  "IO8_FT 166MHz HSLV low speed @ 2.5V"
io8_166m_hslv_ft_ls_pu_2v5  "IO8_FT 166MHz HSLV low speed @ 2.5V pullup"
io8_166m_hslv_ft_ls_pd_2v5  "IO8_FT 166MHz HSLV low speed @ 2.5V pulldown"
[Model Selector] io8_spi_hslv_ft
io8_spi_ft_hs_1v2  "IO8_FT SPI high speed @ 1.2V"
io8_spi_ft_hs_pu_1v2  "IO8_FT SPI high speed @ 1.2V pullup"
io8_spi_ft_hs_pd_1v2  "IO8_FT SPI high speed @ 1.2V pulldown"
io8_spi_ft_fs_1v2  "IO8_FT SPI fast speed @ 1.2V"
io8_spi_ft_fs_pu_1v2  "IO8_FT SPI fast speed @ 1.2V pullup"
io8_spi_ft_fs_pd_1v2  "IO8_FT SPI fast speed @ 1.2V pulldown"
io8_spi_ft_ms_1v2  "IO8_FT SPI med speed @ 1.2V"
io8_spi_ft_ms_pu_1v2  "IO8_FT SPI med speed @ 1.2V pullup"
io8_spi_ft_ms_pd_1v2  "IO8_FT SPI med speed @ 1.2V pulldown"
io8_spi_ft_ls_1v2  "IO8_FT SPI low speed @ 1.2V"
io8_spi_ft_ls_pu_1v2  "IO8_FT SPI low speed @ 1.2V pullup"
io8_spi_ft_ls_pd_1v2  "IO8_FT SPI low speed @ 1.2V pulldown"
io8_spi_ft_hs_1v8  "IO8_FT SPI high speed @ 1.8V"
io8_spi_ft_hs_pu_1v8  "IO8_FT SPI high speed @ 1.8V pullup"
io8_spi_ft_hs_pd_1v8  "IO8_FT SPI high speed @ 1.8V pulldown"
io8_spi_ft_fs_1v8  "IO8_FT SPI fast speed @ 1.8V"
io8_spi_ft_fs_pu_1v8  "IO8_FT SPI fast speed @ 1.8V pullup"
io8_spi_ft_fs_pd_1v8  "IO8_FT SPI fast speed @ 1.8V pulldown"
io8_spi_ft_ms_1v8  "IO8_FT SPI med speed @ 1.8V"
io8_spi_ft_ms_pu_1v8  "IO8_FT SPI med speed @ 1.8V pullup"
io8_spi_ft_ms_pd_1v8  "IO8_FT SPI med speed @ 1.8V pulldown"
io8_spi_ft_ls_1v8  "IO8_FT SPI low speed @ 1.8V"
io8_spi_ft_ls_pu_1v8  "IO8_FT SPI low speed @ 1.8V pullup"
io8_spi_ft_ls_pd_1v8  "IO8_FT SPI low speed @ 1.8V pulldown"
io8_spi_ft_hs_3v3  "IO8_FT SPI high speed @ 3.3V"
io8_spi_ft_hs_pu_3v3  "IO8_FT SPI high speed @ 3.3V pullup"
io8_spi_ft_hs_pd_3v3  "IO8_FT SPI high speed @ 3.3V pulldown"
io8_spi_ft_fs_3v3  "IO8_FT SPI fast speed @ 3.3V"
io8_spi_ft_fs_pu_3v3  "IO8_FT SPI fast speed @ 3.3V pullup"
io8_spi_ft_fs_pd_3v3  "IO8_FT SPI fast speed @ 3.3V pulldown"
io8_spi_ft_ms_3v3  "IO8_FT SPI med speed @ 3.3V"
io8_spi_ft_ms_pu_3v3  "IO8_FT SPI med speed @ 1.8V pullup"
io8_spi_ft_ms_pd_3v3  "IO8_FT SPI med speed @ 3.3V pulldown"
io8_spi_ft_ls_3v3  "IO8_FT SPI low speed @ 3.3V"
io8_spi_ft_ls_pu_3v3  "IO8_FT SPI low speed @ 3.3V pullup"
io8_spi_ft_ls_pd_3v3  "IO8_FT SPI low speed @ 3.3V pulldown"
io8_spi_hslv_ft_hs_1v2  "IO8_FT SPI HSLV high speed @ 1.2V"
io8_spi_hslv_ft_hs_pu_1v2  "IO8_FT SPI HSLV high speed @ 1.2V pullup"
io8_spi_hslv_ft_hs_pd_1v2  "IO8_FT SPI HSLV high speed @ 1.2V pulldown"
io8_spi_hslv_ft_fs_1v2  "IO8_FT SPI HSLV fast speed @ 1.2V"
io8_spi_hslv_ft_fs_pu_1v2  "IO8_FT SPI HSLV fast speed @ 1.2V pullup"
io8_spi_hslv_ft_fs_pd_1v2  "IO8_FT SPI HSLV fast speed @ 1.2V pulldown"
io8_spi_hslv_ft_ms_1v2  "IO8_FT SPI HSLV med speed @ 1.2V"
io8_spi_hslv_ft_ms_pu_1v2  "IO8_FT SPI HSLV med speed @ 1.2V pullup"
io8_spi_hslv_ft_ms_pd_1v2  "IO8_FT SPI HSLV med speed @ 1.2V pulldown"
io8_spi_hslv_ft_ls_1v2  "IO8_FT SPI HSLV low speed @ 1.2V"
io8_spi_hslv_ft_ls_pu_1v2  "IO8_FT SPI HSLV low speed @ 1.2V pullup"
io8_spi_hslv_ft_ls_pd_1v2  "IO8_FT SPI HSLV low speed @ 1.2V pulldown"
io8_spi_hslv_ft_hs_1v8  "IO8_FT SPI HSLV high speed @ 1.8V"
io8_spi_hslv_ft_hs_pu_1v8  "IO8_FT SPI HSLV high speed @ 1.8V pullup"
io8_spi_hslv_ft_hs_pd_1v8  "IO8_FT SPI HSLV high speed @ 1.8V pulldown"
io8_spi_hslv_ft_fs_1v8  "IO8_FT SPI HSLV fast speed @ 1.8V"
io8_spi_hslv_ft_fs_pu_1v8  "IO8_FT SPI HSLV fast speed @ 1.8V pullup"
io8_spi_hslv_ft_fs_pd_1v8  "IO8_FT SPI HSLV fast speed @ 1.8V pulldown"
io8_spi_hslv_ft_ms_1v8  "IO8_FT SPI HSLV med speed @ 1.8V"
io8_spi_hslv_ft_ms_pu_1v8  "IO8_FT SPI HSLV med speed @ 1.8V pullup"
io8_spi_hslv_ft_ms_pd_1v8  "IO8_FT SPI HSLV med speed @ 1.8V pulldown"
io8_spi_hslv_ft_ls_1v8  "IO8_FT SPI HSLV low speed @ 1.8V"
io8_spi_hslv_ft_ls_pu_1v8  "IO8_FT SPI HSLV low speed @ 1.8V pullup"
io8_spi_hslv_ft_ls_pd_1v8  "IO8_FT SPI HSLV low speed @ 1.8V pulldown"
io8_spi_hslv_ft_hs_2v5  "IO8_FT SPI HSLV high speed @ 2.5V"
io8_spi_hslv_ft_hs_pu_2v5  "IO8_FT SPI HSLV high speed @ 2.5V pullup"
io8_spi_hslv_ft_hs_pd_2v5  "IO8_FT SPI HSLV high speed @ 2.5V pulldown"
io8_spi_hslv_ft_fs_2v5  "IO8_FT SPI HSLV fast speed @ 2.5V"
io8_spi_hslv_ft_fs_pu_2v5  "IO8_FT SPI HSLV fast speed @ 2.5V pullup"
io8_spi_hslv_ft_fs_pd_2v5  "IO8_FT SPI HSLV fast speed @ 2.5V pulldown"
io8_spi_hslv_ft_ms_2v5  "IO8_FT SPI HSLV med speed @ 2.5V"
io8_spi_hslv_ft_ms_pu_2v5  "IO8_FT SPI HSLV med speed @ 2.5V pullup"
io8_spi_hslv_ft_ms_pd_2v5  "IO8_FT SPI HSLV med speed @ 2.5V pulldown"
io8_spi_hslv_ft_ls_2v5  "IO8_FT SPI HSLV low speed @ 2.5V"
io8_spi_hslv_ft_ls_pu_2v5  "IO8_FT SPI HSLV low speed @ 2.5V pullup"
io8_spi_hslv_ft_ls_pd_2v5  "IO8_FT SPI HSLV low speed @ 2.5V pulldown"
[Model Selector] io8_spi_ft
io8_spi_ft_hs_1v2  "IO8_FT SPI high speed @ 1.2V"
io8_spi_ft_hs_pu_1v2  "IO8_FT SPI high speed @ 1.2V pullup"
io8_spi_ft_hs_pd_1v2  "IO8_FT SPI high speed @ 1.2V pulldown"
io8_spi_ft_fs_1v2  "IO8_FT SPI fast speed @ 1.2V"
io8_spi_ft_fs_pu_1v2  "IO8_FT SPI fast speed @ 1.2V pullup"
io8_spi_ft_fs_pd_1v2  "IO8_FT SPI fast speed @ 1.2V pulldown"
io8_spi_ft_ms_1v2  "IO8_FT SPI med speed @ 1.2V"
io8_spi_ft_ms_pu_1v2  "IO8_FT SPI med speed @ 1.2V pullup"
io8_spi_ft_ms_pd_1v2  "IO8_FT SPI med speed @ 1.2V pulldown"
io8_spi_ft_ls_1v2  "IO8_FT SPI low speed @ 1.2V"
io8_spi_ft_ls_pu_1v2  "IO8_FT SPI low speed @ 1.2V pullup"
io8_spi_ft_ls_pd_1v2  "IO8_FT SPI low speed @ 1.2V pulldown"
io8_spi_ft_hs_1v8  "IO8_FT SPI high speed @ 1.8V"
io8_spi_ft_hs_pu_1v8  "IO8_FT SPI high speed @ 1.8V pullup"
io8_spi_ft_hs_pd_1v8  "IO8_FT SPI high speed @ 1.8V pulldown"
io8_spi_ft_fs_1v8  "IO8_FT SPI fast speed @ 1.8V"
io8_spi_ft_fs_pu_1v8  "IO8_FT SPI fast speed @ 1.8V pullup"
io8_spi_ft_fs_pd_1v8  "IO8_FT SPI fast speed @ 1.8V pulldown"
io8_spi_ft_ms_1v8  "IO8_FT SPI med speed @ 1.8V"
io8_spi_ft_ms_pu_1v8  "IO8_FT SPI med speed @ 1.8V pullup"
io8_spi_ft_ms_pd_1v8  "IO8_FT SPI med speed @ 1.8V pulldown"
io8_spi_ft_ls_1v8  "IO8_FT SPI low speed @ 1.8V"
io8_spi_ft_ls_pu_1v8  "IO8_FT SPI low speed @ 1.8V pullup"
io8_spi_ft_ls_pd_1v8  "IO8_FT SPI low speed @ 1.8V pulldown"
io8_spi_ft_hs_3v3  "IO8_FT SPI high speed @ 3.3V"
io8_spi_ft_hs_pu_3v3  "IO8_FT SPI high speed @ 3.3V pullup"
io8_spi_ft_hs_pd_3v3  "IO8_FT SPI high speed @ 3.3V pulldown"
io8_spi_ft_fs_3v3  "IO8_FT SPI fast speed @ 3.3V"
io8_spi_ft_fs_pu_3v3  "IO8_FT SPI fast speed @ 3.3V pullup"
io8_spi_ft_fs_pd_3v3  "IO8_FT SPI fast speed @ 3.3V pulldown"
io8_spi_ft_ms_3v3  "IO8_FT SPI med speed @ 3.3V"
io8_spi_ft_ms_pu_3v3  "IO8_FT SPI med speed @ 1.8V pullup"
io8_spi_ft_ms_pd_3v3  "IO8_FT SPI med speed @ 3.3V pulldown"
io8_spi_ft_ls_3v3  "IO8_FT SPI low speed @ 3.3V"
io8_spi_ft_ls_pu_3v3  "IO8_FT SPI low speed @ 3.3V pullup"
io8_spi_ft_ls_pd_3v3  "IO8_FT SPI low speed @ 3.3V pulldown"
io8_spi_hslv_ft_hs_1v2  "IO8_FT SPI HSLV high speed @ 1.2V"
io8_spi_hslv_ft_hs_pu_1v2  "IO8_FT SPI HSLV high speed @ 1.2V pullup"
io8_spi_hslv_ft_hs_pd_1v2  "IO8_FT SPI HSLV high speed @ 1.2V pulldown"
io8_spi_hslv_ft_fs_1v2  "IO8_FT SPI HSLV fast speed @ 1.2V"
io8_spi_hslv_ft_fs_pu_1v2  "IO8_FT SPI HSLV fast speed @ 1.2V pullup"
io8_spi_hslv_ft_fs_pd_1v2  "IO8_FT SPI HSLV fast speed @ 1.2V pulldown"
io8_spi_hslv_ft_ms_1v2  "IO8_FT SPI HSLV med speed @ 1.2V"
io8_spi_hslv_ft_ms_pu_1v2  "IO8_FT SPI HSLV med speed @ 1.2V pullup"
io8_spi_hslv_ft_ms_pd_1v2  "IO8_FT SPI HSLV med speed @ 1.2V pulldown"
io8_spi_hslv_ft_ls_1v2  "IO8_FT SPI HSLV low speed @ 1.2V"
io8_spi_hslv_ft_ls_pu_1v2  "IO8_FT SPI HSLV low speed @ 1.2V pullup"
io8_spi_hslv_ft_ls_pd_1v2  "IO8_FT SPI HSLV low speed @ 1.2V pulldown"
io8_spi_hslv_ft_hs_1v8  "IO8_FT SPI HSLV high speed @ 1.8V"
io8_spi_hslv_ft_hs_pu_1v8  "IO8_FT SPI HSLV high speed @ 1.8V pullup"
io8_spi_hslv_ft_hs_pd_1v8  "IO8_FT SPI HSLV high speed @ 1.8V pulldown"
io8_spi_hslv_ft_fs_1v8  "IO8_FT SPI HSLV fast speed @ 1.8V"
io8_spi_hslv_ft_fs_pu_1v8  "IO8_FT SPI HSLV fast speed @ 1.8V pullup"
io8_spi_hslv_ft_fs_pd_1v8  "IO8_FT SPI HSLV fast speed @ 1.8V pulldown"
io8_spi_hslv_ft_ms_1v8  "IO8_FT SPI HSLV med speed @ 1.8V"
io8_spi_hslv_ft_ms_pu_1v8  "IO8_FT SPI HSLV med speed @ 1.8V pullup"
io8_spi_hslv_ft_ms_pd_1v8  "IO8_FT SPI HSLV med speed @ 1.8V pulldown"
io8_spi_hslv_ft_ls_1v8  "IO8_FT SPI HSLV low speed @ 1.8V"
io8_spi_hslv_ft_ls_pu_1v8  "IO8_FT SPI HSLV low speed @ 1.8V pullup"
io8_spi_hslv_ft_ls_pd_1v8  "IO8_FT SPI HSLV low speed @ 1.8V pulldown"
io8_spi_hslv_ft_hs_2v5  "IO8_FT SPI HSLV high speed @ 2.5V"
io8_spi_hslv_ft_hs_pu_2v5  "IO8_FT SPI HSLV high speed @ 2.5V pullup"
io8_spi_hslv_ft_hs_pd_2v5  "IO8_FT SPI HSLV high speed @ 2.5V pulldown"
io8_spi_hslv_ft_fs_2v5  "IO8_FT SPI HSLV fast speed @ 2.5V"
io8_spi_hslv_ft_fs_pu_2v5  "IO8_FT SPI HSLV fast speed @ 2.5V pullup"
io8_spi_hslv_ft_fs_pd_2v5  "IO8_FT SPI HSLV fast speed @ 2.5V pulldown"
io8_spi_hslv_ft_ms_2v5  "IO8_FT SPI HSLV med speed @ 2.5V"
io8_spi_hslv_ft_ms_pu_2v5  "IO8_FT SPI HSLV med speed @ 2.5V pullup"
io8_spi_hslv_ft_ms_pd_2v5  "IO8_FT SPI HSLV med speed @ 2.5V pulldown"
io8_spi_hslv_ft_ls_2v5  "IO8_FT SPI HSLV low speed @ 2.5V"
io8_spi_hslv_ft_ls_pu_2v5  "IO8_FT SPI HSLV low speed @ 2.5V pullup"
io8_spi_hslv_ft_ls_pd_2v5  "IO8_FT SPI HSLV low speed @ 2.5V pulldown"
[Define Package Model]  481-wlcsp-150-2rdl-dsi-220915
[Manufacturer]  Unknown
[OEM]  Unknown
[Description]  None
[Number Of Pins]  132
[Pin Numbers]
| Pin Num   Terminal Name
L13 | DSI_CKN
J13 | DSI_CKP
G13 | DSI_D0N
E13 | DSI_D0P
R13 | DSI_D1N
N13 | DSI_D1P
U11 | NRST
W11 | PA0
V10 | PA1
R9 | PA2
N9 | PA3
M8 | PA4
AA11 | PA5
U9 | PA6
P8 | PA7
H4 | PA8
F2 | PA9
G3 | PA10
E1 | PA11
C1 | PA12
E3 | PA13
F4 | PA14
B4 | PA15
Y10 | PB0
W9 | PB1
M6 | PB2
B8 | PB3
E7 | PB4
A9 | PB5
D8 | PB6
G7 | PB7
C9 | PB8
F8 | PB9
W5 | PB10
AA5 | PB11
AA3 | PB12
Y4 | PB13
V4 | PB14
Y2 | PB15
P10 | PC0
L7 | PC1
Y12 | PC2
T10 | PC3
T8 | PC4
N7 | PC5
N5 | PC6
J3 | PC7
K4 | PC8
L5 | PC9
D4 | PC10
J5 | PC11
A5 | PC12
E11 | PC13
A13 | PC14-OSC32_IN
B12 | PC15-OSC32_OUT
C5 | PD0
E5 | PD1
G5 | PD2
K6 | PD3
B6 | PD4
D6 | PD5
F6 | PD6
H6 | PD7
W3 | PD8
U3 | PD9
W1 | PD10
R3 | PD11
T2 | PD12
N3 | PD13
P2 | PD14
R1 | PD15
H8 | PE0
E9 | PE1
D10 | PE2
G9 | PE3
J9 | PE4
F10 | PE5
D12 | PE6
T6 | PE7
AA7 | PE8
V6 | PE9
R5 | PE10
U5 | PE11
Y6 | PE12
AB6 | PE13
P4 | PE14
T4 | PE15
G11 | PF0
H10 | PF1
F12 | PF2
L11 | PF3
N11 | PF4
R11 | PF5
J11 | PF6
K10 | PF7
M10 | PF8
L9 | PF9
K8 | PF10
R7 | PF11
V8 | PF12
AA9 | PF13
Y8 | PF14
U7 | PF15
P6 | PG0
W7 | PG1
N1 | PG2
L1 | PG3
M2 | PG4
L3 | PG5
M4 | PG6
J1 | PG7
K2 | PG8
W13 | PH0-OSC_IN
V12 | PH1-OSC_OUT
J7 | PH3-BOOT0
AB2 | VDD11
B10 | VDD11
B2 | VDD11
C13 | VBAT
A3 | VDD
H12 | VDDDSI
M12 | VDD11DSI
A1 | VDDUSB
AC13 | VDDA
G1 | VDDIO2
AB4 | VDDSMPS
AC5 | VLXSMPS
AB12 | VREFP
AA1 | VSS
K12 | VSSDSI
AA13 | VSSA_VREFM
AC3 | VSSSMPS
|[Merged Pins]  A3
|A7  |  VDD
|A11  |  VDD
|AC1  |  VDD
|AC7  |  VDD
|AC9  |  VDD
|AC11  |  VDD
|U1  |  VDD
|U13  |  VDD
|[Merged Pins]  AA1
|AB8  |  VSS
|AB10  |  VSS
|C3  |  VSS
|C7  |  VSS
|C11  |  VSS
|D2  |  VSS
|H2  |  VSS
|T12  |  VSS
|V2  |  VSS
|[Merged Pins]  K12
|P12  |  VSS_DSI
[Model Data]
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[End Model Data]
[End Package Model]
| Models and submodels in the file (265): io8_100m_ft_hs_1v2 (I/O), io8_100m_ft_hs_pu_1v2 (I/O), io8_100m_ft_hs_pd_1v2 (I/O), io8_100m_ft_fs_1v2 (I/O), io8_100m_ft_fs_pu_1v2 (I/O), io8_100m_ft_fs_pd_1v2 (I/O), io8_100m_ft_ms_1v2 (I/O), io8_100m_ft_ms_pu_1v2 (I/O), io8_100m_ft_ms_pd_1v2 (I/O), io8_100m_ft_ls_1v2 (I/O), io8_100m_ft_ls_pu_1v2 (I/O), io8_100m_ft_ls_pd_1v2 (I/O), io8_100m_ft_hs_1v8 (I/O), io8_100m_ft_hs_pu_1v8 (I/O), io8_100m_ft_hs_pd_1v8 (I/O), io8_100m_ft_fs_1v8 (I/O), io8_100m_ft_fs_pu_1v8 (I/O), io8_100m_ft_fs_pd_1v8 (I/O), io8_100m_ft_ms_1v8 (I/O), io8_100m_ft_ms_pu_1v8 (I/O), io8_100m_ft_ms_pd_1v8 (I/O), io8_100m_ft_ls_1v8 (I/O), io8_100m_ft_ls_pu_1v8 (I/O), io8_100m_ft_ls_pd_1v8 (I/O), io8_100m_ft_hs_3v3 (I/O), io8_100m_ft_hs_pu_3v3 (I/O), io8_100m_ft_hs_pd_3v3 (I/O), io8_100m_ft_fs_3v3 (I/O), io8_100m_ft_fs_pu_3v3 (I/O), io8_100m_ft_fs_pd_3v3 (I/O), io8_100m_ft_ms_3v3 (I/O), io8_100m_ft_ms_pu_3v3 (I/O), io8_100m_ft_ms_pd_3v3 (I/O), io8_100m_ft_ls_3v3 (I/O), io8_100m_ft_ls_pu_3v3 (I/O), io8_100m_ft_ls_pd_3v3 (I/O), io8_100m_hslv_ft_hs_1v2 (I/O), io8_100m_hslv_ft_hs_pu_1v2 (I/O), io8_100m_hslv_ft_hs_pd_1v2 (I/O), io8_100m_hslv_ft_fs_1v2 (I/O), io8_100m_hslv_ft_fs_pu_1v2 (I/O), io8_100m_hslv_ft_fs_pd_1v2 (I/O), io8_100m_hslv_ft_ms_1v2 (I/O), io8_100m_hslv_ft_ms_pu_1v2 (I/O), io8_100m_hslv_ft_ms_pd_1v2 (I/O), io8_100m_hslv_ft_ls_1v2 (I/O), io8_100m_hslv_ft_ls_pu_1v2 (I/O), io8_100m_hslv_ft_ls_pd_1v2 (I/O), io8_100m_hslv_ft_hs_1v8 (I/O), io8_100m_hslv_ft_hs_pu_1v8 (I/O), io8_100m_hslv_ft_hs_pd_1v8 (I/O), io8_100m_hslv_ft_fs_1v8 (I/O), io8_100m_hslv_ft_fs_pu_1v8 (I/O), io8_100m_hslv_ft_fs_pd_1v8 (I/O), io8_100m_hslv_ft_ms_1v8 (I/O), io8_100m_hslv_ft_ms_pu_1v8 (I/O), io8_100m_hslv_ft_ms_pd_1v8 (I/O), io8_100m_hslv_ft_ls_1v8 (I/O), io8_100m_hslv_ft_ls_pu_1v8 (I/O), io8_100m_hslv_ft_ls_pd_1v8 (I/O), io8_100m_hslv_ft_hs_2v5 (I/O), io8_100m_hslv_ft_hs_pu_2v5 (I/O), io8_100m_hslv_ft_hs_pd_2v5 (I/O), io8_100m_hslv_ft_fs_2v5 (I/O), io8_100m_hslv_ft_fs_pu_2v5 (I/O), io8_100m_hslv_ft_fs_pd_2v5 (I/O), io8_100m_hslv_ft_ms_2v5 (I/O), io8_100m_hslv_ft_ms_pu_2v5 (I/O), io8_100m_hslv_ft_ms_pd_2v5 (I/O), io8_100m_hslv_ft_ls_2v5 (I/O), io8_100m_hslv_ft_ls_pu_2v5 (I/O), io8_100m_hslv_ft_ls_pd_2v5 (I/O), io8_100m_i2c_ft_1v2 (I/O_open_drain), io8_100m_i2c_ft_pu_1v2 (I/O_open_drain), io8_100m_i2c_ft_pd_1v2 (I/O_open_drain), io8_100m_i2c_ft_1v8 (I/O_open_drain), io8_100m_i2c_ft_pu_1v8 (I/O_open_drain), io8_100m_i2c_ft_pd_1v8 (I/O_open_drain), io8_100m_i2c_ft_3v3 (I/O_open_drain), io8_100m_i2c_ft_pu_3v3 (I/O_open_drain)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
